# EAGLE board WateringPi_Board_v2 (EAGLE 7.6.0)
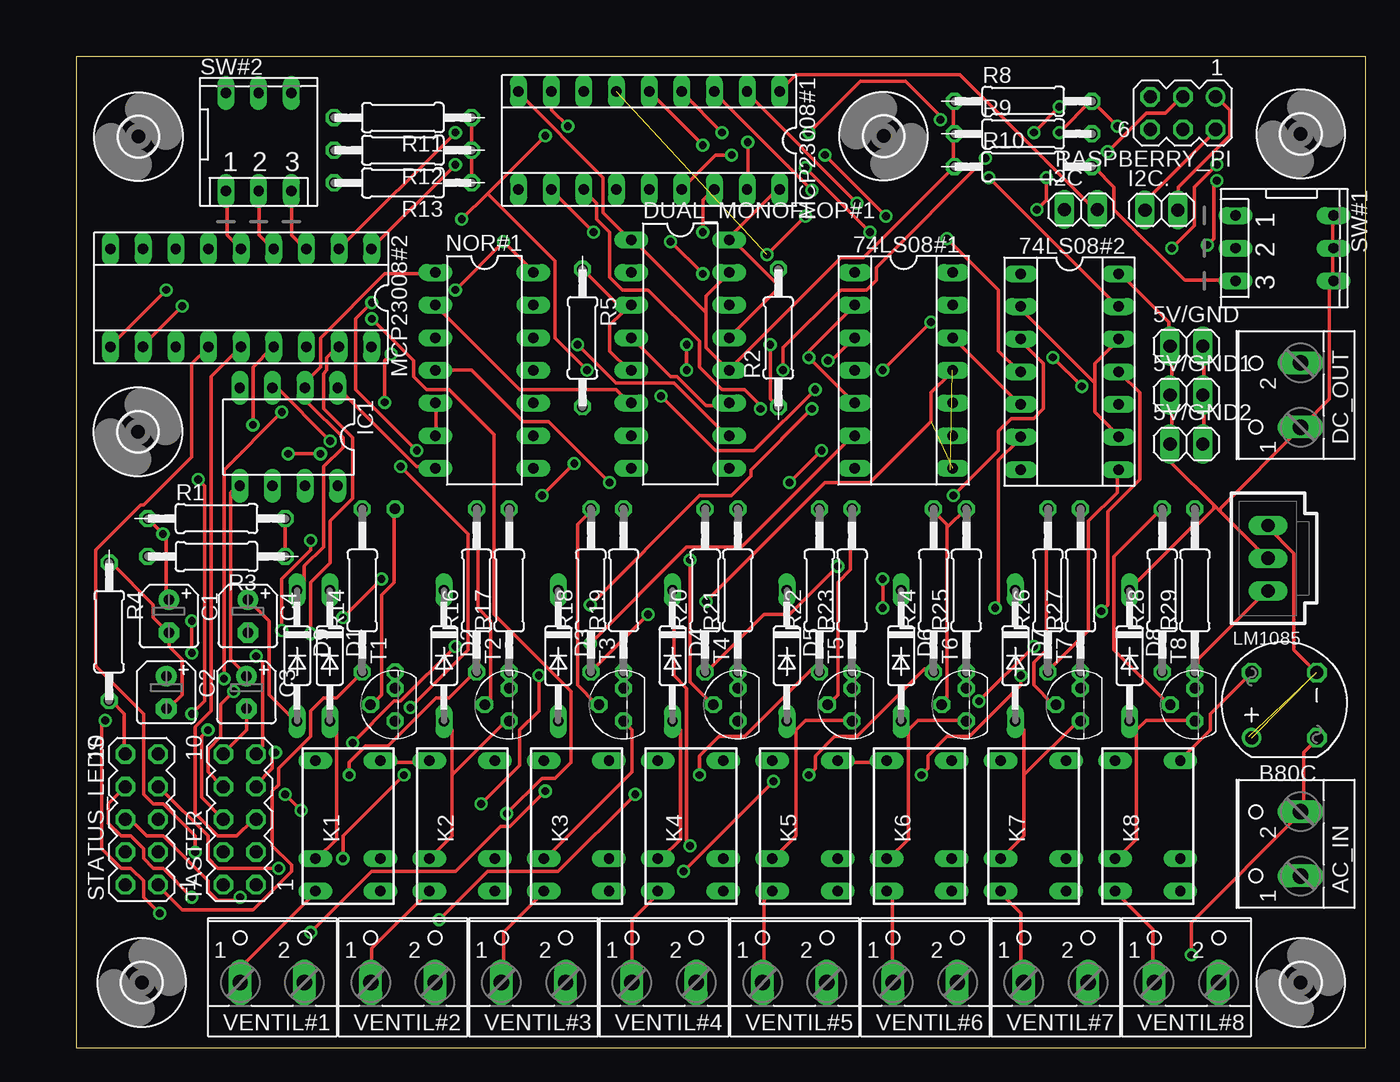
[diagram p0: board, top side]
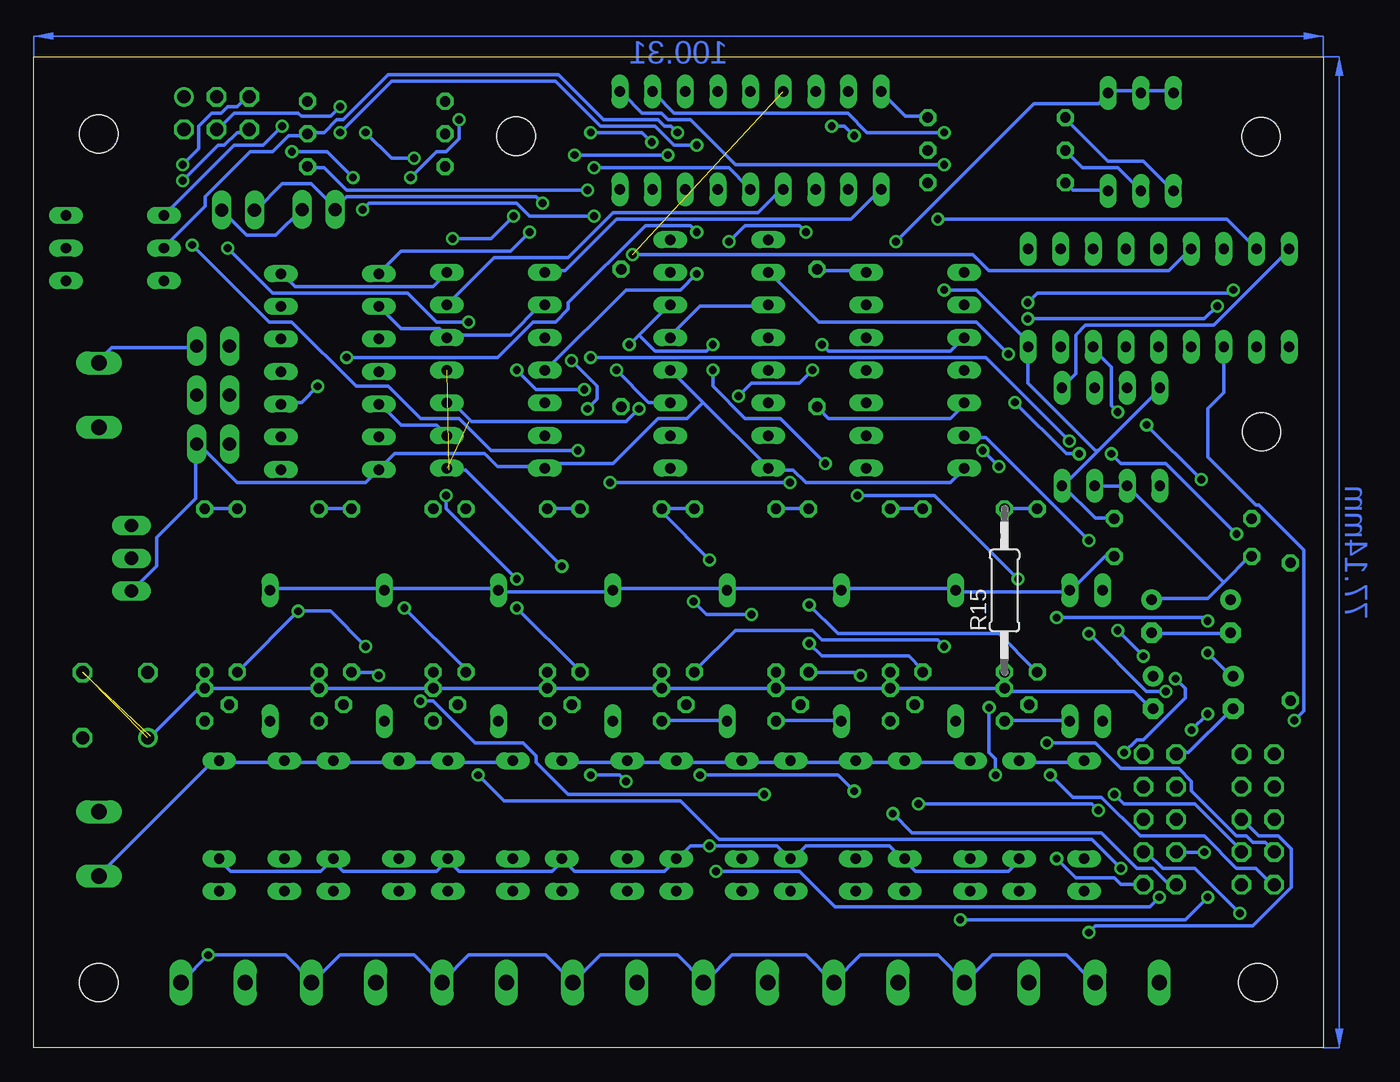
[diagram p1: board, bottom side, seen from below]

Size 100.31 x 77.14 mm. Coordinates in mm from the lower left corner, seen from the top.
Outline: 0,0 100.31,0 100.31,77.14 0,77.14 0,0
Copper layers (1*16): Top 0.035mm / dielectric 1.5mm / Bottom 0.035mm
Design rules "default": minimum track width 10mil, minimum drill 24mil, track to track 8mil, track to pad 8mil, pad to pad 8mil, via to via 8mil, smd to smd 8mil, copper to edge 40mil, drill to drill 8mil, minimum pad ring 10mil, minimum via ring 8mil, stop-mask expansion 4mil, vias tented up to drill 0mil, thermal gap 10mil

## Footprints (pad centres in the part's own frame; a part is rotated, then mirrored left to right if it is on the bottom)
1X02 = drill 1.016 long: 1 -1.27,0; 2 1.27,0
SOCKET-14 = drill 0.813 long: 1 -7.62,-3.81; 2 -5.08,-3.81; 3 -2.54,-3.81; 4 0,-3.81; 5 2.54,-3.81; 6 5.08,-3.81; 7 7.62,-3.81; 8 7.62,3.81; 9 5.08,3.81; 10 2.54,3.81; 11 0,3.81; 12 -2.54,3.81; 13 -5.08,3.81; 14 -7.62,3.81
W237-102 = drill 1.194 long: 1 -2.5,-1.27; 2 2.5,-1.27
RB1A = drill 1.016: + -2.54,2.54 | drill 1.016 octagon: - 2.54,-2.54; AC1 2.54,2.54; AC2 -2.54,-2.54
B45181A = drill 0.813 pad 1.6: + -1.27,0 | drill 0.813 pad 1.6 octagon: - 1.27,0
DO35-10 = drill 0.813 long: A 5.08,0; C -5.08,0
DIL16 = drill 0.813 long: 1 -8.89,-3.81; 2 -6.35,-3.81; 3 -3.81,-3.81; 4 -1.27,-3.81; 5 1.27,-3.81; 6 3.81,-3.81; 7 6.35,-3.81; 8 8.89,-3.81; 9 8.89,3.81; 10 6.35,3.81; 11 3.81,3.81; 12 1.27,3.81; 13 -1.27,3.81; 14 -3.81,3.81; 15 -6.35,3.81; 16 -8.89,3.81
3,0 = hole 3: 0,0
DIL-08 = drill 0.813 long: 1 -3.81,-3.81; 2 -1.27,-3.81; 3 1.27,-3.81; 4 3.81,-3.81; 5 3.81,3.81; 6 1.27,3.81; 7 -1.27,3.81; 8 -3.81,3.81
G5V1 = drill 0.813 long: 1 -5.08,-2.54; 2 -2.54,-2.54; 5 5.08,-2.54; 6 5.08,2.54; 9 -2.54,2.54; 10 -5.08,2.54
70543-03 = drill 1.016 long: 1 -2.54,0; 2 0,0; 3 2.54,0
SOCKET-18 = drill 0.813 long: 1 -10.16,-3.81; 2 -7.62,-3.81; 3 -5.08,-3.81; 4 -2.54,-3.81; 5 0,-3.81; 6 2.54,-3.81; 7 5.08,-3.81; 8 7.62,-3.81; 9 10.16,-3.81; 10 10.16,3.81; 11 7.62,3.81; 12 5.08,3.81; 13 2.54,3.81; 14 0,3.81; 15 -2.54,3.81; 16 -5.08,3.81; 17 -7.62,3.81; 18 -10.16,3.81
DIL14 = drill 0.813 long: 1 -7.62,-3.81; 2 -5.08,-3.81; 3 -2.54,-3.81; 4 0,-3.81; 5 2.54,-3.81; 6 5.08,-3.81; 7 7.62,-3.81; 8 7.62,3.81; 9 5.08,3.81; 10 2.54,3.81; 11 0,3.81; 12 -2.54,3.81; 13 -5.08,3.81; 14 -7.62,3.81
9/1 = drill 0.813 octagon: 1 -5.35,0; 2 5.35,0
0207/12 = drill 0.813 octagon: 1 -6.35,0; 2 6.35,0
MA03-2 = drill 1.016: 1 -2.54,-1.27 | drill 1.016 octagon: 2 -2.54,1.27; 3 0,-1.27; 4 0,1.27; 5 2.54,-1.27; 6 2.54,1.27
MA05-2 = drill 1.016 octagon: 1 -5.08,-1.27; 2 -5.08,1.27; 3 -2.54,-1.27; 4 -2.54,1.27; 5 0,-1.27; 6 0,1.27; 7 2.54,-1.27; 8 2.54,1.27; 9 5.08,-1.27; 10 5.08,1.27
DP-03 = drill 0.813 long: 1 -2.54,-3.81; 2 0,-3.81; 3 2.54,-3.81; 4 2.54,3.81; 5 0,3.81; 6 -2.54,3.81
TO92 = drill 0.813 octagon: 1 1.27,0; 2 0,1.905; 3 -1.27,0

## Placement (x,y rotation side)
5V/GND  [1X02]  86.36,54.61 0 top
5V/GND1  [1X02]  86.36,50.8 0 top
5V/GND2  [1X02]  86.36,46.99 0 top
74LS08#1  [SOCKET-14]  64.36,52.72 270 top
74LS08#2  [SOCKET-14]  77.26,52.62 270 top
AC_IN  [W237-102]  93.98,15.88 90 top
B80C  RECTIFIER-RB1A  [RB1A]  93.98,26.67 90 top
C1  10uF  [B45181A]  7.19,33.59 270 top
C2  10uF  [B45181A]  6.99,27.65 270 top
C3  10nF  [B45181A]  13.23,27.65 270 top
C4  10uF  [B45181A]  13.34,33.59 270 top
D1  1N4148DO35-10  [DO35-10]  19.7,30.52 270 top
D2  1N4148DO35-10  [DO35-10]  28.59,30.52 270 top
D3  1N4148DO35-10  [DO35-10]  37.48,30.52 270 top
D4  1N4148DO35-10  [DO35-10]  46.37,30.52 270 top
D5  1N4148DO35-10  [DO35-10]  55.26,30.52 270 top
D6  1N4148DO35-10  [DO35-10]  64.15,30.52 270 top
D7  1N4148DO35-10  [DO35-10]  73.04,30.52 270 top
D8  1N4148DO35-10  [DO35-10]  81.93,30.52 270 top
D9  1N4148DO35-10  [DO35-10]  17.16,30.52 270 top
DC_OUT  [W237-102]  93.98,50.8 90 top
DUAL_MONOFLOP#1  4538N  [DIL16]  46.99,53.99 270 top
H1  RPI-HOLE3.0  [3,0]  4.83,70.91 0 top
H2  RPI-HOLE3.0  [3,0]  62.8,70.94 270 top
H5  MOUNT-HOLE3.0  [3,0]  4.78,47.94 0 top
H6  MOUNT-HOLE3.0  [3,0]  5.08,5.08 0 top
H7  MOUNT-HOLE3.0  [3,0]  95.25,71.12 0 top
H8  MOUNT-HOLE3.0  [3,0]  95.25,5.08 0 top
I2C  [1X02]  78.15,65.24 0 top
I2C.  [1X02]  84.41,65.2 0 top
IC1  NE555  [DIL-08]  16.51,47.54 180 top
K1  G5V1  [G5V1]  21.12,17.27 90 top
K2  G5V1  [G5V1]  30.01,17.27 90 top
K3  G5V1  [G5V1]  38.9,17.27 90 top
K4  G5V1  [G5V1]  47.79,17.27 90 top
K5  G5V1  [G5V1]  56.68,17.27 90 top
K6  G5V1  [G5V1]  65.57,17.27 90 top
K7  G5V1  [G5V1]  74.46,17.27 90 top
K8  G5V1  [G5V1]  83.35,17.27 90 top
LM1085  C-GRID-03-70543  [70543-03]  92.71,38.1 90 top
MCP23008#1  [SOCKET-18]  44.55,70.61 180 top
MCP23008#2  [SOCKET-18]  12.8,58.35 180 top
NOR#1  7402N  [DIL14]  31.75,52.72 270 top
R1  1M  [9/1]  10.9,41.19 0 top
R2  1M  [9/1]  54.61,55.24 90 top
R3  1M  [9/1]  10.9,38.24 180 top
R4  Null Ohm  [9/1]  2.54,32.38 270 top
R5  1M  [9/1]  39.37,55.24 270 top
R8  1M  [9/1]  73.66,73.66 0 top
R9  1M  [9/1]  73.66,71.12 0 top
R10  1M  [9/1]  73.66,68.58 0 top
R11  1M  [9/1]  25.4,72.39 180 top
R12  1M  [9/1]  25.4,69.85 180 top
R13  1M  [9/1]  25.4,67.31 180 top
R14  2,2k  [0207/12]  22.24,35.6 90 top
R15  2,2k  [0207/12]  24.78,35.6 90 bottom
R16  2,2k  [0207/12]  31.13,35.6 90 top
R17  2,2k  [0207/12]  33.67,35.6 90 top
R18  2,2k  [0207/12]  40.02,35.6 90 top
R19  2,2k  [0207/12]  42.56,35.6 90 top
R20  2,2k  [0207/12]  48.91,35.6 90 top
R21  2,2k  [0207/12]  51.45,35.6 90 top
R22  2,2k  [0207/12]  57.8,35.6 90 top
R23  2,2k  [0207/12]  60.34,35.6 90 top
R24  2,2k  [0207/12]  66.69,35.6 90 top
R25  2,2k  [0207/12]  69.23,35.6 90 top
R26  2,2k  [0207/12]  75.58,35.6 90 top
R27  2,2k  [0207/12]  78.12,35.6 90 top
R28  2,2k  [0207/12]  84.47,35.6 90 top
R29  2,2k  [0207/12]  87.01,35.6 90 top
RASPBERRY_PI  [MA03-2]  86.09,72.74 180 top
STATUS_LEDS  [MA05-2]  5.08,17.78 90 top
SW#1  [DP-03]  93.98,62.23 270 top
SW#2  [DP-03]  14.18,70.5 0 top
T1  BC337  [TO92]  24.78,26.71 90 top
T2  BC337  [TO92]  33.67,26.71 90 top
T3  BC337  [TO92]  42.56,26.71 90 top
T4  BC337  [TO92]  51.45,26.71 90 top
T5  BC337  [TO92]  60.34,26.71 90 top
T6  BC337  [TO92]  69.23,26.71 90 top
T7  BC337  [TO92]  78.12,26.71 90 top
T8  BC337  [TO92]  87.01,26.71 90 top
TASTER  [MA05-2]  12.7,17.78 90 top
VENTIL#1  [W237-102]  15.24,6.35 0 top
VENTIL#2  [W237-102]  25.4,6.35 0 top
VENTIL#3  [W237-102]  35.56,6.35 0 top
VENTIL#4  [W237-102]  45.72,6.35 0 top
VENTIL#5  [W237-102]  55.88,6.35 0 top
VENTIL#6  [W237-102]  66.04,6.35 0 top
VENTIL#7  [W237-102]  76.2,6.35 0 top
VENTIL#8  [W237-102]  86.36,6.35 0 top

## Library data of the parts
5V/GND 5V/GND1 5V/GND2 I2C I2C. = pinhead
74LS08#1 74LS08#2 MCP23008#1 MCP23008#2 = ic-package
AC_IN DC_OUT VENTIL#1-VENTIL#8 = con-wago-500; MPN: 237-102; OC_FARNELL: unknown; OC_NEWARK: 70K9898
B80C = rectifier
C1-C4 R14-R29 = resistor
D1-D9 = diode
DUAL_MONOFLOP#1 = 45xx
H1 H2 H5-H8 = holes
IC1 = st-microelectronics; MF: Arrow Electronics; MPN: NE555N; OC_FARNELL: 1467742; OC_NEWARK: 89K1486
K1-K8 = relay
LM1085 = con-molex; OC_FARNELL: unknown; OC_NEWARK: unknown
NOR#1 = 74ttl-din
R1-R5 R8-R13 = customize
RASPBERRY_PI STATUS_LEDS TASTER = con-lstb; OC_FARNELL: unknown; OC_NEWARK: unknown
SW#1 SW#2 = switch-dil; MPN: MCDP03; OC_FARNELL: 1522004; OC_NEWARK: 74M2976
T1-T8 = transistor

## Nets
+5V: 5V/GND1.1 5V/GND2.1 5V/GND.1 74LS08#1.14 74LS08#2.14 D1.C D2.C D3.C D4.C D5.C D6.C D7.C D8.C DC_OUT.1 DUAL_MONOFLOP#1.3 DUAL_MONOFLOP#1.5 DUAL_MONOFLOP#1.13 DUAL_MONOFLOP#1.16 IC1.4 IC1.8 K1.2 K2.2 K3.2 K4.2 K5.2 K6.2 K7.2 K8.2 LM1085.2 MCP23008#1.18 MCP23008#2.18 NOR#1.14 R1.2 R2.2 R3.1 R5.1 SW#1.4 SW#1.5 SW#1.6 SW#2.4 SW#2.5 SW#2.6
AC_1/2: AC_IN.1 B80C.AC1 K1.5 K1.6 K2.5 K2.6 K3.5 K3.6 K4.5 K4.6 K5.5 K5.6 K6.5 K6.6 K7.5 K7.6 K8.5 K8.6
AC_2/2: AC_IN.2 B80C.AC2 VENTIL#1.2 VENTIL#2.2 VENTIL#3.2 VENTIL#4.2 VENTIL#5.2 VENTIL#6.2 VENTIL#7.2 VENTIL#8.2
GND: 5V/GND1.2 5V/GND2.2 5V/GND.2 74LS08#1.7 74LS08#2.7 B80C.- C1.- C2.- C3.- C4.- DC_OUT.2 DUAL_MONOFLOP#1.1 DUAL_MONOFLOP#1.8 DUAL_MONOFLOP#1.12 DUAL_MONOFLOP#1.15 IC1.1 LM1085.1 MCP23008#1.9 MCP23008#2.9 NOR#1.7 R4.1 R8.1 R9.1 R10.1 R11.1 R12.1 R13.1 R15.1 R17.1 R19.1 R21.1 R23.1 R25.1 R27.1 R29.1 T1.1 T2.1 T3.1 T4.1 T5.1 T6.1 T7.1 T8.1 TASTER.10
I2C_SCL: I2C.2 I2C..2 MCP23008#1.1 MCP23008#2.1 RASPBERRY_PI.1
I2C_SDA: I2C.1 I2C..1 MCP23008#1.2 MCP23008#2.2 RASPBERRY_PI.2
INTERRUPT: MCP23008#2.8 RASPBERRY_PI.5
IS_ALIVE: D9.C IC1.2 NOR#1.1
KEEP_ALIVE: DUAL_MONOFLOP#1.4 DUAL_MONOFLOP#1.11 RASPBERRY_PI.4
MCP23008#1_A0: MCP23008#1.5 R8.2 SW#1.1
MCP23008#1_A1: MCP23008#1.4 R9.2 SW#1.2
MCP23008#1_A2: MCP23008#1.3 R10.2 SW#1.3
MCP23008#1_OUT0: 74LS08#1.1 MCP23008#1.10
MCP23008#1_OUT1: 74LS08#1.4 MCP23008#1.11
MCP23008#1_OUT2: 74LS08#1.10 MCP23008#1.12
MCP23008#1_OUT3: 74LS08#1.13 MCP23008#1.13
MCP23008#1_OUT4: 74LS08#2.1 MCP23008#1.14
MCP23008#1_OUT5: 74LS08#2.4 MCP23008#1.15
MCP23008#1_OUT6: 74LS08#2.10 MCP23008#1.16
MCP23008#1_OUT7: 74LS08#2.13 MCP23008#1.17
MCP23008#2_A0: MCP23008#2.5 R11.2 SW#2.1
MCP23008#2_A1: MCP23008#2.4 R12.2 SW#2.2
MCP23008#2_A2: MCP23008#2.3 R13.2 SW#2.3
MCP_RESET: MCP23008#1.6 MCP23008#2.6 RASPBERRY_PI.3
N$1: R14.2 R15.2 T1.2
N$2: C2.+ DUAL_MONOFLOP#1.14 R2.1
N$3: C1.+ DUAL_MONOFLOP#1.2 R1.1
N$4: DUAL_MONOFLOP#1.10 NOR#1.3
N$5: DUAL_MONOFLOP#1.6 NOR#1.2
N$6: R16.2 R17.2 T2.2
N$7: C3.+ IC1.5
N$8: D1.A K1.9 T1.3
N$9: D2.A K2.9 T2.3
N$10: R18.2 R19.2 T3.2
N$11: D3.A K3.9 T3.3
N$12: B80C.+ LM1085.3
N$13: R20.2 R21.2 T4.2
N$14: R4.2 STATUS_LEDS.10
N$15: C4.+ D9.A IC1.6 IC1.7 R3.2
N$22: D4.A K4.9 T4.3
N$23: R22.2 R23.2 T5.2
N$24: D5.A K5.9 T5.3
N$25: R24.2 R25.2 T6.2
N$26: D6.A K6.9 T6.3
N$27: R26.2 R27.2 T7.2
N$28: D7.A K7.9 T7.3
N$29: R28.2 R29.2 T8.2
N$30: D8.A K8.9 T8.3
NOTAUS: NOR#1.4 RASPBERRY_PI.6
NOTAUS_RAW: NOR#1.5 NOR#1.6 R5.2 TASTER.9
RELAIS#1_ENABLE: 74LS08#1.3 R14.1 STATUS_LEDS.1
RELAIS#1_OUT: K1.10 VENTIL#1.1
RELAIS#2_ENABLE: 74LS08#1.6 R16.1 STATUS_LEDS.2
RELAIS#2_OUT: K2.10 VENTIL#2.1
RELAIS#3_ENABLE: 74LS08#1.8 R18.1 STATUS_LEDS.3
RELAIS#3_OUT: K3.10 VENTIL#3.1
RELAIS#4_ENABLE: 74LS08#1.11 R20.1 STATUS_LEDS.4
RELAIS#4_OUT: K4.10 VENTIL#4.1
RELAIS#5_ENABLE: 74LS08#2.3 R22.1 STATUS_LEDS.5
RELAIS#5_OUT: K5.10 VENTIL#5.1
RELAIS#6_ENABLE: 74LS08#2.6 R24.1 STATUS_LEDS.6
RELAIS#6_OUT: K6.10 VENTIL#6.1
RELAIS#7_ENABLE: 74LS08#2.8 R26.1 STATUS_LEDS.7
RELAIS#7_OUT: K7.10 VENTIL#7.1
RELAIS#8_ENABLE: 74LS08#2.11 R28.1 STATUS_LEDS.8
RELAIS#8_OUT: K8.10 VENTIL#8.1
RPI_STILL_ALIVE: 74LS08#1.2 74LS08#1.5 74LS08#1.9 74LS08#1.12 74LS08#2.2 74LS08#2.5 74LS08#2.9 74LS08#2.12 IC1.3
TASTE#1: MCP23008#2.10 TASTER.1
TASTE#2: MCP23008#2.11 TASTER.2
TASTE#3: MCP23008#2.12 TASTER.3
TASTE#4: MCP23008#2.13 TASTER.4
TASTE#5: MCP23008#2.14 TASTER.5
TASTE#6: MCP23008#2.15 TASTER.6
TASTE#7: MCP23008#2.16 TASTER.7
TASTE#8: MCP23008#2.17 TASTER.8

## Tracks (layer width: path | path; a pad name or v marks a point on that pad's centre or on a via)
+5V  (via drill 0.61)
  Top 0.254: 54.48,59.48 54.48,60.48 R2.2 | 54.48,59.48 54.48,58.98 50.98,55.48 DUAL_MONOFLOP#1.13 | 54.48,59.48 50.98,62.98 | 50.98,62.98 50.98,63.23 54.48,66.73 MCP23008#1.18 | 50.98,62.98 DUAL_MONOFLOP#1.16 | 42.48,57.23 42.98,57.73 DUAL_MONOFLOP#1.3 42.48,57.23 | 42.48,57.23 41.48,56.23 41.48,54.23 42.98,52.73 DUAL_MONOFLOP#1.5 | 42.48,57.23 42.48,57.48 39.48,60.48 R5.1 | NOR#1.14 35.48,60.48 v33.23,62.73 v29.48,58.98 | 74LS08#2.14 81.23,60.23 84.98,56.48 84.98,54.73 5V/GND.1 85.23,54.48 85.23,50.98 5V/GND1.1 85.23,50.73 85.23,47.23 5V/GND2.1 85.23,46.98 85.23,45.48 88.48,42.23 | 97.73,62.23 97.73,59.73 SW#1.4 97.73,59.48 97.48,59.23 97.48,50.48 95.48,48.48 DC_OUT.1 95.23,48.23 88.98,41.98 88.98,41.73 | 97.73,62.23 97.73,64.73 SW#1.6 | 97.73,62.23 SW#1.5 | 88.48,42.23 88.98,41.73 | 88.98,41.73 92.48,38.23 LM1085.2 | 88.48,42.23 88.48,41.98 87.23,40.73 86.98,40.73 81.98,35.73 D8.C | R1.2 16.23,40.98 16.23,38.48 R3.1 | v47.73,15.73 47.48,15.98 47.48,27.98 46.48,28.98 46.48,35.48 D4.C
  Bottom 0.254: SW#2.6 11.73,74.48 13.98,74.48 SW#2.5 14.23,74.48 16.48,74.48 SW#2.4 16.73,74.23 17.48,73.48 22.48,73.48 v33.23,62.73 | NOR#1.14 35.73,60.48 39.23,60.48 R5.1 | DUAL_MONOFLOP#1.13 50.73,55.48 48.48,57.73 43.23,57.73 DUAL_MONOFLOP#1.3 | K1.2 23.73,14.48 24.48,13.73 31.73,13.73 32.48,14.48 K2.2 32.73,14.73 33.73,15.73 40.23,15.73 41.23,14.73 K3.2 41.48,14.73 42.48,15.73 v47.73,15.73 49.23,15.73 50.23,14.73 K4.2 50.48,14.48 51.23,13.73 58.23,13.73 58.98,14.48 K5.2 59.23,14.48 59.98,13.73 67.23,13.73 67.98,14.48 K6.2 68.23,14.48 68.98,13.73 76.23,13.73 76.98,14.48 K7.2 77.23,14.48 77.98,13.73 84.98,13.73 85.73,14.48 K8.2 | 74LS08#1.14 68.23,60.23 69.23,59.23 79.98,59.23 80.98,60.23 74LS08#2.14 | D8.C 81.73,35.73 73.23,35.73 D7.C 72.98,35.73 64.23,35.73 D6.C 63.98,35.48 55.48,35.48 D5.C 55.23,35.73 46.48,35.73 D4.C 46.23,35.73 37.73,35.73 D3.C 37.48,35.73 28.73,35.73 D2.C 28.48,35.48 19.73,35.48 D1.C 19.48,35.73 16.98,38.23 16.48,38.23 R3.1 | R1.2 16.48,41.23 17.73,41.23 20.23,43.73 IC1.8 20.23,43.98 19.98,43.98 17.48,46.48 | 17.48,46.48 12.73,51.23 IC1.4 | 17.48,46.48 17.73,46.48 22.98,51.73 22.98,54.48 MCP23008#2.18 22.73,54.73 26.98,58.98 v29.48,58.98
AC_1/2
  Top 0.254: B80C.AC1 91.23,28.98 88.23,25.98 88.23,24.73 85.98,22.48 K8.5 | K2.6 27.23,22.23 23.73,22.23 K1.5 | K5.5 59.23,22.23 62.98,22.23 K6.6
  Bottom 0.254: AC_IN.1 95.23,13.48 86.48,22.23 85.98,22.23 K8.5 85.73,22.23 80.98,22.23 K8.6 80.73,22.23 77.23,22.23 K7.5 76.98,22.23 71.98,22.23 K7.6 71.73,22.23 68.23,22.23 K6.5 67.98,22.23 63.23,22.23 K6.6 | K1.6 18.73,22.23 23.48,22.23 K1.5 | K5.5 58.98,22.23 54.23,22.23 K5.6 53.98,22.23 50.48,22.23 K4.5 50.23,22.23 45.48,22.23 K4.6 45.23,22.23 41.48,22.23 K3.5 41.23,22.23 36.48,22.23 K3.6 36.23,22.23 32.73,22.23 K2.5 32.48,22.23 27.48,22.23 K2.6
AC_2/2  (via drill 0.61)
  Top 0.254: B80C.AC2 96.48,23.98 95.48,22.98 95.48,18.48 AC_IN.2 95.23,18.23 86.73,9.73 v86.73,7.23
  Bottom 0.254: VENTIL#1.2 17.98,5.23 19.98,7.23 25.73,7.23 27.73,5.23 VENTIL#2.2 27.98,5.23 29.98,7.23 35.98,7.23 37.98,5.23 VENTIL#3.2 38.23,5.23 40.23,7.23 45.98,7.23 47.98,5.23 VENTIL#4.2 48.23,5.23 50.23,7.23 56.23,7.23 VENTIL#5.2 58.48,5.23 60.48,7.23 66.48,7.23 68.48,5.23 VENTIL#6.2 68.73,5.23 70.73,7.23 76.48,7.23 78.48,5.23 VENTIL#7.2 78.73,5.23 80.73,7.23 v86.73,7.23 88.73,5.23 VENTIL#8.2
GND  (1 unrouted)
  Top 0.254: NOR#1.7 27.73,45.23 26.48,45.23 20.48,51.23 IC1.1 | R13.1 30.73,67.48 30.73,69.73 R12.1 30.73,69.98 30.73,72.23 R11.1 | R8.1 68.23,73.48 68.23,71.23 R9.1 68.23,70.98 68.23,68.73 R10.1 68.23,68.48 61.23,61.48 59.48,61.48 50.98,52.98 50.98,52.73 DUAL_MONOFLOP#1.12 50.73,52.73 48.98,54.48 48.98,57.23 | 48.98,57.23 48.98,58.48 50.73,60.23 DUAL_MONOFLOP#1.15 | 48.98,57.23 43.23,62.98 DUAL_MONOFLOP#1.1 42.98,62.98 40.98,64.98 40.98,67.73 34.48,74.23 MCP23008#1.9 | TASTER.10 11.48,22.98 13.23,24.73 13.23,26.23 C3.- | R4.1 2.73,37.73 5.98,34.48 5.98,33.48 6.98,32.48 C1.- 7.23,32.23 7.23,31.23 8.23,30.23 8.23,27.48 7.23,26.48 C2.- | T1.1 24.73,27.98 24.73,29.23 R15.1 | T2.1 33.73,27.98 33.73,29.23 R17.1 | T3.1 42.48,27.98 42.48,29.23 R19.1 | T4.1 51.48,27.98 51.48,29.23 R21.1 | T7.1 78.23,27.98 78.23,29.23 R27.1 | T5.1 60.48,27.98 60.48,29.23 R23.1 | T6.1 69.23,29.23 R25.1 | 5V/GND2.2 87.73,47.23 87.73,50.73 5V/GND1.2 87.73,50.98 87.73,54.48 5V/GND.2 | T8.1 86.98,27.98 86.98,29.23 R29.1 87.23,29.48 87.23,30.23 92.48,35.48 LM1085.1
  Bottom 0.254: MCP23008#2.9 2.73,61.98 8.48,56.23 18.48,56.23 19.23,55.48 19.23,52.48 20.23,51.48 IC1.1 | MCP23008#1.9 34.23,74.23 32.48,72.48 30.98,72.48 R11.1 | 48.23,50.23 50.48,52.48 50.73,52.48 DUAL_MONOFLOP#1.12 | 48.23,50.23 43.23,45.23 DUAL_MONOFLOP#1.8 42.98,44.98 41.23,44.98 40.23,43.98 28.98,43.98 27.98,44.98 NOR#1.7 | 48.23,50.23 49.48,48.98 51.73,48.98 55.23,45.48 60.23,45.48 60.48,45.23 74LS08#1.7 60.73,45.23 64.23,45.23 65.23,46.23 72.23,46.23 73.23,45.23 74LS08#2.7 73.48,44.98 74.48,43.98 84.48,43.98 87.48,46.98 5V/GND2.2 87.73,46.98 87.73,42.73 90.73,39.73 90.73,37.48 92.48,35.73 LM1085.1 | C2.- 7.23,26.23 10.48,22.98 11.23,22.98 TASTER.10 | C4.- 13.23,32.23 7.23,32.23 C1.- | C3.- 13.48,26.48 14.73,27.73 24.73,27.73 T1.1 24.98,27.98 33.48,27.98 T2.1 33.73,27.98 42.48,27.98 T3.1 42.73,27.98 51.23,27.98 T4.1 51.48,27.98 60.23,27.98 T5.1 60.48,27.98 T6.1 69.48,27.98 77.98,27.98 T7.1 78.23,27.98 86.98,27.98 T8.1 87.23,27.73 87.73,27.73 91.23,24.23 | DC_OUT.2 95.23,53.48 94.23,54.48 87.73,54.48 5V/GND.2
I2C_SCL  (via drill 0.61)
  Top 0.254: RASPBERRY_PI.1 88.73,73.98 89.73,72.98 89.73,70.98 85.73,66.98 85.73,65.23 I2C..2 | v29.48,68.73 22.98,62.23 MCP23008#2.1 | I2C.2 79.23,65.23 68.73,75.73 55.98,75.73 54.73,74.48 MCP23008#1.1
  Bottom 0.254: I2C..2 85.48,64.98 83.73,63.23 81.48,63.23 79.48,65.23 I2C.2 | v29.48,68.73 45.73,68.73 49.23,72.23 50.98,72.23 51.48,72.73 52.98,72.73 54.48,74.23 MCP23008#1.1
I2C_SDA  (via drill 0.61)
  Top 0.254: RASPBERRY_PI.2 88.48,71.23 83.23,65.98 83.23,65.23 I2C..1 | v29.48,71.23 20.48,62.23 MCP23008#2.2 | v60.73,65.73 52.23,74.23 MCP23008#1.2
  Bottom 0.254: I2C..1 82.98,65.23 80.98,67.23 78.73,67.23 76.98,65.48 I2C.1 76.73,65.48 75.98,66.23 61.23,66.23 v60.73,65.73 | v29.48,71.23 35.48,71.23 36.98,72.73 50.48,72.73 51.98,74.23 MCP23008#1.2
INTERRUPT  (via drill 0.61)
  Top 0.254: v36.48,70.98 31.98,66.48 | 31.98,66.48 v29.98,64.48 | v38.23,71.73 36.98,72.98 36.98,74.23 | v88.73,68.73 86.98,66.98 86.98,63.98 v85.23,62.23 | v62.73,52.73 v66.48,56.48 | v57.48,51.23 52.73,46.48 49.73,46.48 v45.48,50.73 | v39.73,52.73 37.23,55.23 37.23,61.23 31.98,66.48
  Bottom 0.254: v29.98,64.48 7.48,64.48 5.23,62.23 MCP23008#2.8 | v36.48,70.98 37.23,71.73 v38.23,71.73 | v88.73,68.73 87.48,69.98 87.48,71.73 86.48,72.73 85.73,72.73 85.23,73.23 84.48,73.23 83.73,73.98 RASPBERRY_PI.5 | v85.23,62.23 81.73,58.73 71.23,58.73 68.98,56.48 v66.48,56.48 | v62.73,52.73 61.23,51.23 v57.48,51.23 | v45.48,50.73 44.48,51.73 40.73,51.73 v39.73,52.73
IS_ALIVE
  Top 0.254: D9.C 17.23,35.73 17.73,36.23 17.73,37.48 19.23,38.98 19.23,45.23 20.73,46.73 20.73,47.48 17.98,50.23 17.98,51.23 IC1.2 17.98,51.48 17.98,51.98 18.98,52.98 18.98,55.23 23.98,60.23 27.73,60.23 NOR#1.1
KEEP_ALIVE  (via drill 0.61)
  Top 0.254: DUAL_MONOFLOP#1.4 43.23,55.23 46.23,52.23 46.73,52.23 48.98,49.98 50.73,49.98 DUAL_MONOFLOP#1.11 | v74.48,71.23 v76.48,73.23 | v70.73,69.23 62.23,60.73 62.23,59.73 61.48,58.98 59.48,58.98 54.98,54.48 v54.98,52.73
  Bottom 0.254: v76.48,73.23 77.23,72.48 79.48,72.48 79.73,72.73 84.73,72.73 85.98,71.48 RASPBERRY_PI.4 | v74.48,71.23 72.48,69.23 v70.73,69.23 | v54.98,52.73 52.48,50.23 50.98,50.23 DUAL_MONOFLOP#1.11
MCP23008#1_A0  (via drill 0.61)
  Top 0.254: v48.73,70.23 44.73,74.23 MCP23008#1.5 | v76.48,71.23 78.98,73.73 R8.2 79.23,73.48 v80.98,71.73
  Bottom 0.254: v48.73,70.23 50.48,70.23 51.98,71.73 56.23,71.73 59.73,75.23 72.48,75.23 v76.48,71.23 | v80.98,71.73 82.48,70.23 84.73,70.23 89.98,64.98 SW#1.1
MCP23008#1_A1  (via drill 0.61)
  Top 0.254: v50.23,71.23 47.23,74.23 MCP23008#1.4
  Bottom 0.254: v50.23,71.23 50.73,71.73 51.23,71.73 51.73,72.23 55.98,72.23 59.48,75.73 72.73,75.73 76.23,72.23 76.73,72.23 77.73,71.23 78.98,71.23 R9.2 79.23,70.98 80.48,70.98 81.73,69.73 83.48,69.73 86.98,66.23 86.98,65.48 90.23,62.23 SW#1.2
MCP23008#1_A2  (via drill 0.61)
  Top 0.254: v57.23,66.73 49.73,74.23 MCP23008#1.3 | SW#1.3 89.98,59.73 86.23,59.73 80.73,65.23 80.73,66.98 79.23,68.48 R10.2
  Bottom 0.254: v57.23,66.73 75.98,66.73 77.73,68.48 78.98,68.48 R10.2
MCP23008#1_OUT0
  Bottom 0.254: MCP23008#1.10 34.48,66.73 36.73,64.48 54.98,64.48 58.98,60.48 60.48,60.48 74LS08#1.1
MCP23008#1_OUT1  (via drill 0.61)
  Top 0.254: v40.23,63.48 36.98,66.73 MCP23008#1.11 | v48.73,60.23 v46.23,62.73
  Bottom 0.254: v40.23,63.48 40.73,63.98 44.98,63.98 v46.23,62.73 | v48.73,60.23 49.98,58.98 54.23,58.98 60.48,52.73 74LS08#1.4
MCP23008#1_OUT2  (via drill 0.61)
  Top 0.254: v53.23,49.73 53.23,49.98 51.98,51.23 50.23,51.23 48.48,52.98 48.48,54.98 44.48,58.98 42.48,58.98 41.48,59.98 41.48,63.48 40.48,64.48 40.48,65.73 39.48,66.73 MCP23008#1.12
  Bottom 0.254: v53.23,49.73 54.23,48.73 66.23,48.73 67.48,49.98 67.98,49.98 74LS08#1.10
MCP23008#1_OUT3
  Bottom 0.254: MCP23008#1.13 42.23,66.73 43.98,64.98 55.23,64.98 58.73,61.48 64.48,61.48 67.98,57.98 74LS08#1.13
MCP23008#1_OUT4  (via drill 0.61)
  Top 0.254: v61.73,63.48 v56.73,68.48
  Bottom 0.254: v56.73,68.48 46.23,68.48 44.73,66.98 MCP23008#1.14 | v61.73,63.48 63.23,61.98 71.73,61.98 73.23,60.48 74LS08#2.1
MCP23008#1_OUT5  (via drill 0.61)
  Top 0.254: v50.98,69.48 49.73,69.48 47.23,66.98 MCP23008#1.15 | v62.98,64.73 v58.23,69.48 | v67.73,62.98 71.73,58.98 71.73,54.23 73.23,52.73 74LS08#2.4
  Bottom 0.254: v58.23,69.48 v50.98,69.48 | v62.98,64.73 64.73,62.98 v67.73,62.98
MCP23008#1_OUT6  (via drill 0.61)
  Top 0.254: v48.73,63.48 48.73,65.98 49.48,66.73 MCP23008#1.16 | v78.23,51.48 v75.98,53.73
  Bottom 0.254: v48.73,63.48 49.23,63.98 52.73,63.98 58.73,57.98 58.73,57.48 59.73,56.48 61.48,56.48 64.23,53.73 v75.98,53.73 | v78.23,51.48 79.48,50.23 80.98,50.23 74LS08#2.10
MCP23008#1_OUT7  (via drill 0.61)
  Top 0.254: v52.23,70.48 52.23,66.98 MCP23008#1.17 | v56.98,71.23 60.98,75.23 64.48,75.23 67.23,72.48 v67.23,72.23 | v70.98,67.73 80.98,57.73 74LS08#2.13
  Bottom 0.254: v52.23,70.48 52.98,71.23 v56.98,71.23 | v67.23,72.23 67.23,70.73 68.23,69.73 68.98,69.73 v70.98,67.73
MCP23008#2_A0
  Top 0.254: MCP23008#2.5 12.73,62.23 11.73,63.23 11.73,66.48 SW#2.1
  Bottom 0.254: R11.2 19.98,72.23 16.73,68.98 13.98,68.98 11.73,66.73 SW#2.1
MCP23008#2_A1
  Top 0.254: MCP23008#2.4 15.23,62.23 14.23,63.23 14.23,66.48 SW#2.2
  Bottom 0.254: R12.2 19.98,69.73 18.73,68.48 15.98,68.48 14.23,66.73 SW#2.2
MCP23008#2_A2
  Top 0.254: MCP23008#2.3 17.73,62.23 16.73,63.23 16.73,66.48 SW#2.3
  Bottom 0.254: R13.2 19.98,67.23 19.48,66.73 16.73,66.73 SW#2.3
MCP_RESET  (via drill 0.61)  (1 unrouted)
  Top 0.254: v56.73,64.73 v53.73,61.73 | v74.73,65.23 75.48,65.98 v75.48,67.73 | v80.23,69.73 83.23,72.73 84.73,72.73 85.98,73.98 RASPBERRY_PI.3
  Bottom 0.254: v53.73,61.73 27.23,61.73 25.98,60.48 11.98,60.48 10.48,61.98 MCP23008#2.6 | v56.73,64.73 61.73,64.73 62.73,65.73 74.23,65.73 v74.73,65.23 | v75.48,67.73 77.48,69.73 v80.23,69.73
N$1
  Top 0.254: T1.2 22.98,26.73 23.73,27.48 23.73,35.23 24.73,36.23 24.73,41.73 R15.2
  Bottom 0.254: R14.2 22.48,41.98 24.73,41.98 R15.2
N$2  (via drill 0.61)
  Top 0.254: v53.98,54.73 53.98,50.48 54.48,49.98 R2.1 | v8.98,33.23 v8.98,30.73 | v23.73,36.48 v20.73,33.48 | v38.73,45.48 v36.23,42.98 | v47.48,54.73 v47.48,52.73
  Bottom 0.254: v53.98,54.73 53.23,55.48 | 53.23,55.48 50.98,57.73 DUAL_MONOFLOP#1.14 | v8.98,30.73 7.23,28.98 C2.+ | v8.98,33.23 9.23,33.48 v20.73,33.48 | v23.73,36.48 30.23,42.98 v36.23,42.98 | v38.73,45.48 42.23,48.98 44.98,48.98 47.48,51.48 v47.48,52.73 | v47.48,54.73 47.98,54.23 51.98,54.23 53.23,55.48
N$3  (via drill 0.61)
  Top 0.254: R1.1 5.73,40.98 v6.73,39.98 6.98,39.73 6.98,34.98 C1.+ | v24.48,53.98 23.98,53.48 v23.98,50.23 | v16.48,46.23 v18.98,46.23
  Bottom 0.254: v24.48,53.98 26.98,56.48 39.23,56.48 42.98,60.23 DUAL_MONOFLOP#1.2 | v23.98,50.23 19.98,46.23 v18.98,46.23 | v16.48,46.23 15.73,45.48 12.23,45.48 v6.73,39.98
N$4  (via drill 0.61)
  Top 0.254: v38.98,54.73 41.98,51.73 46.48,51.73 50.73,47.48 DUAL_MONOFLOP#1.10
  Bottom 0.254: v38.98,54.73 38.48,54.23 28.98,54.23 27.98,55.23 NOR#1.3
N$5
  Top 0.254: NOR#1.2 27.98,57.73 34.48,51.23 41.98,51.23 42.98,50.23 DUAL_MONOFLOP#1.6
N$6
  Top 0.254: T2.2 31.98,26.73 32.23,26.98 32.23,33.23 31.23,34.23 31.23,41.73 R16.2
  Bottom 0.254: R17.2 33.48,41.98 31.23,41.98 R16.2
N$7
  Top 0.254: IC1.5 12.48,43.73 11.98,43.23 11.98,30.23 13.23,28.98 C3.+
N$8
  Top 0.254: K1.9 18.73,14.73 20.23,16.23 20.23,24.73 19.73,25.23 D1.A
  Bottom 0.254: T1.3 24.73,25.48 19.73,25.48 D1.A
N$9
  Top 0.254: 29.23,21.23 29.23,24.73 28.73,25.23 D2.A | 29.23,21.23 29.23,16.48 K2.9 | 29.23,21.23 33.48,25.48 T2.3
N$10
  Top 0.254: T3.2 40.48,26.73 38.98,28.23 38.98,40.73 39.98,41.73 R18.2
  Bottom 0.254: R18.2 40.23,41.98 42.48,41.98 R19.2
N$11
  Top 0.254: K3.9 36.48,14.73 43.23,21.48 43.23,24.73 42.73,25.23 T3.3
  Bottom 0.254: D3.A 37.73,25.48 42.48,25.48 T3.3
N$12  (1 unrouted)
  Top 0.254: 96.48,29.23 94.73,30.98 94.73,38.48 92.73,40.48 LM1085.3
N$13  (via drill 0.61)
  Top 0.254: v47.73,37.98 47.73,28.48 49.48,26.73 T4.2
  Bottom 0.254: R20.2 48.98,41.98 51.23,41.98 R21.2 51.48,41.73 v47.73,37.98
N$14
  Top 0.254: R4.2 2.73,26.98 3.73,25.98 3.73,22.98 STATUS_LEDS.10
N$15
  Top 0.254: D9.A 16.98,25.48 14.98,27.48 14.98,33.23 13.48,34.73 C4.+
  Bottom 0.254: IC1.7 17.73,43.73 15.48,43.73 IC1.6 7.73,36.23 | 7.73,36.23 8.98,34.98 13.23,34.98 C4.+ | 7.73,36.23 5.73,38.23 R3.2
N$22
  Top 0.254: K4.9 45.48,14.73 46.98,16.23 46.98,24.73 46.48,25.23 D4.A
  Bottom 0.254: T4.3 51.23,25.48 46.48,25.48 D4.A
N$23
  Top 0.254: T5.2 58.48,26.73 59.23,27.48 59.23,36.23 60.23,37.23 60.23,41.73 R23.2
  Bottom 0.254: R22.2 57.98,41.98 60.23,41.98 R23.2
N$24
  Top 0.254: 55.98,24.73 55.98,16.48 54.23,14.73 K5.9 | 55.98,24.73 55.48,25.23 D5.A | 55.98,24.73 56.73,25.48 60.23,25.48 T5.3
N$25
  Top 0.254: 67.73,40.48 67.73,40.73 66.73,41.73 R24.2 | 67.73,40.48 67.73,26.98 67.48,26.73 T6.2 | 67.73,40.48 69.23,41.98 R25.2
N$26
  Top 0.254: 64.73,24.73 64.73,16.23 63.23,14.73 K6.9 | 64.73,24.73 64.23,25.23 D6.A 64.73,24.73 | 64.73,24.73 65.48,25.48 69.23,25.48 T6.3
N$27
  Top 0.254: T7.2 75.98,26.73 74.48,28.23 74.48,29.98 75.48,30.98 75.48,41.73 R26.2
  Bottom 0.254: R27.2 77.98,41.98 75.73,41.98 R26.2
N$28
  Top 0.254: 73.73,21.23 73.73,24.73 73.23,25.23 D7.A | 73.73,21.23 73.73,16.48 71.98,14.73 K7.9 | 73.73,21.23 77.98,25.48 T7.3
N$29
  Top 0.254: T8.2 84.98,26.73 80.73,30.98 80.73,38.23 84.23,41.73 R28.2
  Bottom 0.254: R29.2 86.98,41.98 84.48,41.98 R28.2
N$30
  Top 0.254: 82.48,24.73 82.48,16.23 80.98,14.73 K8.9 | 82.48,24.73 81.98,25.23 D8.A 82.48,24.73 | 82.48,24.73 83.23,25.48 86.98,25.48 T8.3
NOTAUS  (via drill 0.61)
  Top 0.254: v41.48,43.98 36.73,48.73 34.73,48.73 30.73,52.73 27.98,52.73 NOR#1.4 | v57.98,46.48 v55.48,43.98 | v87.98,62.48 88.48,62.98 88.48,67.23 v88.73,67.48
  Bottom 0.254: v55.48,43.98 v41.48,43.98 | v57.98,46.48 64.73,46.48 67.23,48.98 70.23,48.98 72.73,51.48 75.23,51.48 80.23,56.48 81.98,56.48 v87.98,62.48 | v88.73,67.48 85.98,70.23 85.48,70.23 84.48,71.23 83.73,71.23 RASPBERRY_PI.6
NOTAUS_RAW  (via drill 0.61)
  Top 0.254: NOR#1.6 27.98,47.73 27.98,49.98 NOR#1.5 | v13.98,30.48 14.48,29.98 14.48,23.48 13.98,22.98 TASTER.9 | v15.98,32.48 15.98,36.48 18.23,38.73 v18.23,39.48
  Bottom 0.254: R5.2 39.23,49.73 38.48,48.98 28.98,48.98 27.98,49.98 NOR#1.5 | v15.98,32.48 v13.98,30.48 | v18.23,39.48 26.23,47.48 27.73,47.48 NOR#1.6
RELAIS#1_ENABLE  (via drill 0.61)
  Top 0.254: R14.1 22.23,29.23 20.23,27.23 19.23,27.23 18.23,26.23 18.23,24.23 15.73,21.73 15.73,20.48 15.23,19.98 15.23,15.73 16.73,14.23 16.73,13.73 13.73,10.73 8.23,10.73 6.48,12.48 STATUS_LEDS.1 | v58.48,53.48 58.73,53.48 60.48,55.23 74LS08#1.3 | v57.23,49.73 52.48,44.98 52.48,44.48 50.98,42.98 48.48,42.98 v39.98,34.48
  Bottom 0.254: v58.48,53.48 56.48,51.48 56.48,50.48 v57.23,49.73 | v39.98,34.48 37.73,32.23 25.23,32.23 22.48,29.48 R14.1
RELAIS#1_OUT
  Top 0.254: K1.10 18.48,11.98 12.98,6.48 12.98,5.23 VENTIL#1.1
RELAIS#2_ENABLE  (via drill 0.61)
  Top 0.254: v21.23,21.23 21.23,22.23 22.48,23.48 24.23,23.48 27.98,27.23 28.98,27.23 30.98,29.23 R16.1 | v39.98,31.48 47.48,38.98 51.73,38.98 60.48,47.73 74LS08#1.6
  Bottom 0.254: v21.23,21.23 19.48,19.48 17.23,19.48 14.23,16.48 9.23,16.48 6.73,13.98 5.23,13.98 3.98,12.73 STATUS_LEDS.2 | v39.98,31.48 38.98,30.48 32.23,30.48 31.23,29.48 R16.1
RELAIS#2_OUT
  Top 0.254: K2.10 27.23,11.98 22.98,7.73 22.98,5.23 VENTIL#2.1
RELAIS#3_ENABLE  (via drill 0.61)  (1 unrouted)
  Top 0.254: v44.48,33.73 40.23,29.48 R18.1 | v48.98,34.73 58.23,43.98 61.73,43.98 66.48,48.73 66.48,50.98 67.98,52.48 | v17.48,18.48 v16.23,19.73 | v31.48,18.98 34.48,21.98 34.48,24.73 35.98,26.23 v35.98,28.98
  Bottom 0.254: v44.48,33.73 47.98,33.73 v48.98,34.73 | v16.23,19.73 15.48,18.98 9.98,18.98 6.48,15.48 STATUS_LEDS.3 | v17.48,18.48 17.98,18.98 v31.48,18.98 | v35.98,28.98 36.23,29.23 39.98,29.23 R18.1
RELAIS#3_OUT
  Top 0.254: K3.10 36.23,11.98 33.23,8.98 33.23,5.23 VENTIL#3.1
RELAIS#4_ENABLE  (via drill 0.61)  (1 unrouted)
  Top 0.254: v59.23,37.48 55.48,33.73 53.48,33.73 48.98,29.23 R20.1 | v21.48,23.73 24.73,26.98 25.23,26.98 v29.48,31.23
  Bottom 0.254: v59.23,37.48 66.73,44.98 67.98,44.98 | v21.48,23.73 17.73,23.73 15.73,21.73 11.23,21.73 10.23,20.73 10.23,19.98 6.73,16.48 5.98,16.48 5.48,15.98 4.48,15.98 3.98,15.48 STATUS_LEDS.4 | v29.48,31.23 29.98,31.73 38.98,31.73 39.73,32.48 45.73,32.48 48.73,29.48 R20.1
RELAIS#4_OUT
  Top 0.254: K4.10 45.23,11.98 43.23,9.98 43.23,5.23 VENTIL#4.1
RELAIS#5_ENABLE  (via drill 0.61)
  Top 0.254: v62.73,36.48 v62.73,34.23 | v68.23,42.98 71.73,46.48 71.73,47.98 72.73,48.98 74.48,48.98 75.23,49.73 75.23,53.23 73.48,54.98 74LS08#2.3 | v18.23,8.98 22.98,13.73 29.48,13.73 32.98,17.23 33.73,17.23 v36.48,19.98 | v48.48,21.23 48.48,22.73 49.98,24.23 51.98,24.23 57.23,29.48 57.73,29.48 R22.1
  Bottom 0.254: v62.73,34.23 57.98,29.48 R22.1 | v62.73,36.48 68.23,41.98 v68.23,42.98 | v18.23,8.98 17.73,9.48 5.48,9.48 2.48,12.48 2.48,15.48 3.48,16.48 4.98,16.48 6.23,17.73 STATUS_LEDS.5 | v36.48,19.98 37.73,21.23 v48.48,21.23
RELAIS#5_OUT
  Top 0.254: K5.10 53.98,11.98 53.48,11.48 53.48,5.23 VENTIL#5.1
RELAIS#6_ENABLE  (via drill 0.61)
  Top 0.254: v71.48,34.23 71.73,34.48 71.73,45.73 73.23,47.23 73.23,47.48 74LS08#2.6 | v12.73,11.73 12.48,11.48 10.98,11.48 10.23,12.23 10.23,12.98 6.73,16.48 5.48,16.48 3.98,17.98 STATUS_LEDS.6 | v54.23,20.73 v47.23,13.73 | v56.98,21.23 57.48,21.73 57.48,22.73 58.98,24.23 60.73,24.23 65.98,29.48 66.48,29.48 R24.1
  Bottom 0.254: v71.48,34.23 66.73,29.48 R24.1 | v12.73,11.73 13.48,10.98 37.98,10.98 40.73,13.73 v47.23,13.73 | v54.23,20.73 54.73,21.23 v56.98,21.23
RELAIS#6_OUT
  Top 0.254: K6.10 63.23,11.98 63.48,11.73 63.48,5.23 VENTIL#6.1
RELAIS#7_ENABLE  (via drill 0.61)
  Top 0.254: R26.1 75.73,29.48 78.73,32.48 78.73,40.98 80.98,43.23 80.98,44.98 74LS08#2.8 | v15.73,13.98 10.98,13.98 10.23,14.73 10.23,16.48 6.48,20.23 STATUS_LEDS.7 | v65.73,21.23 66.23,21.73 66.23,22.73 67.73,24.23 69.48,24.23 73.48,28.23 v73.48,28.98
  Bottom 0.254: v15.73,13.98 17.98,16.23 46.98,16.23 49.98,19.23 63.73,19.23 v65.73,21.23 | v73.48,28.98 73.73,29.23 75.48,29.23 R26.1
RELAIS#7_OUT
  Top 0.254: K7.10 71.98,11.98 73.48,10.48 73.48,5.23 VENTIL#7.1
RELAIS#8_ENABLE  (via drill 0.61)
  Top 0.254: v79.73,33.98 80.23,34.48 80.23,41.73 82.73,44.23 82.73,50.98 81.23,52.48 74LS08#2.11 | v8.98,11.73 6.73,13.98 5.98,13.98 5.23,14.73 5.23,15.48 4.23,16.48 3.48,16.48 2.48,17.48 2.48,18.98 3.73,20.23 STATUS_LEDS.8 | v28.23,9.98 31.98,13.73 37.48,13.73 v43.48,19.73 | v74.48,31.23 v70.23,26.98
  Bottom 0.254: R28.1 84.23,29.48 v79.73,33.98 77.23,33.98 v74.48,31.23 | v8.98,11.73 10.73,9.98 v28.23,9.98 | v43.48,19.73 58.73,19.73 61.23,22.23 61.23,22.73 62.23,23.73 65.98,23.73 69.23,26.98 v70.23,26.98
RELAIS#8_OUT
  Top 0.254: K8.10 80.98,11.98 83.73,9.23 83.73,5.23 VENTIL#8.1
RPI_STILL_ALIVE  (via drill 0.61)
  Top 0.254: 79.23,51.73 79.23,53.23 80.98,54.98 74LS08#2.12 | 79.23,51.73 79.23,49.48 80.98,47.73 74LS08#2.9 | 79.23,51.73 73.48,57.48 74LS08#2.2 | 74LS08#2.5 73.23,50.23 68.23,55.23 74LS08#1.12 | v19.73,47.23 15.48,51.48 IC1.3 | 74LS08#1.5 60.48,50.23 v56.98,53.73 56.98,54.23 60.48,57.73 74LS08#1.2
  Bottom 0.254: 74LS08#1.9 68.23,47.73 68.98,48.48 71.73,48.48 73.23,49.98 74LS08#2.5 | 74LS08#2.2 73.23,57.48 71.73,55.98 68.73,55.98 68.23,55.48 74LS08#1.12 67.98,55.48 63.23,55.48 60.98,57.73 60.73,57.73 74LS08#1.2 | v19.73,47.23 26.23,53.73 v56.98,53.73
TASTE#1  (via drill 0.61)
  Top 0.254: v6.98,58.98 2.73,54.73 MCP23008#2.10 | v22.98,57.98 21.73,56.73 21.73,51.23 v26.48,46.48 | v25.23,45.23 30.48,39.98 30.48,30.98 v25.98,26.48 | v25.48,21.23 20.73,16.48 v20.73,14.73
  Bottom 0.254: v6.98,58.98 7.23,58.73 22.23,58.73 v22.98,57.98 | v25.23,45.23 v26.48,46.48 | v25.98,26.48 25.98,22.98 25.48,22.48 v25.48,21.23 | v20.73,14.73 19.23,13.23 16.23,13.23 15.73,12.73 13.98,12.73 TASTER.1
TASTE#2  (via drill 0.61)
  Top 0.254: v8.23,57.73 5.23,54.73 MCP23008#2.11 | v22.98,56.73 26.23,53.48 26.23,52.23 27.23,51.23 28.98,51.23 32.48,47.73 32.48,33.73 38.48,27.73 38.48,22.23 37.23,20.98 36.23,20.98 v33.48,18.23
  Bottom 0.254: v8.23,57.73 9.23,56.73 v22.98,56.73 | v33.48,18.23 31.98,16.73 17.23,16.73 14.48,13.98 13.23,13.98 11.98,12.73 11.48,12.73 TASTER.2
TASTE#3  (via drill 0.61)
  Top 0.254: v2.23,25.48 1.98,25.23 1.98,15.48 3.48,13.98 4.23,13.98 5.23,12.98 5.23,11.73 v6.48,10.48
  Bottom 0.254: v2.23,25.48 1.48,26.23 1.48,38.73 4.98,42.23 5.23,42.23 8.98,45.98 8.98,49.73 7.73,50.98 7.73,54.48 MCP23008#2.12 | v6.48,10.48 9.98,13.98 12.48,13.98 13.73,15.23 TASTER.3
TASTE#4  (via drill 0.61)
  Top 0.254: v9.23,15.23 9.23,16.48 6.73,18.98 5.98,18.98 5.23,19.73 5.23,25.98 1.48,29.73 1.48,38.73 4.98,42.23 5.23,42.23 8.98,45.98 8.98,53.23 10.23,54.48 MCP23008#2.13
  Bottom 0.254: v9.23,15.23 11.23,15.23 TASTER.4
TASTE#5
  Top 0.254: MCP23008#2.14 12.73,54.48 10.48,52.23 10.48,26.23 9.23,24.98 9.23,18.23 10.98,16.48 12.48,16.48 13.73,17.73 TASTER.5
TASTE#6  (via drill 0.61)
  Top 0.254: v13.73,48.48 13.73,52.98 15.23,54.48 MCP23008#2.15 | v9.48,44.23 9.98,43.73 9.98,26.98 v8.98,25.98 | v10.23,24.73 9.73,24.23 9.73,19.48 TASTER.6
  Bottom 0.254: v9.48,44.23 v13.73,48.48 | v10.23,24.73 v8.98,25.98
TASTE#7  (via drill 0.61)
  Top 0.254: v15.98,49.48 11.48,44.98 v11.48,28.73 | v15.48,22.98 15.23,22.73 15.23,21.73 13.98,20.48 TASTER.7
  Bottom 0.254: v15.98,49.48 16.48,49.98 16.48,52.98 17.98,54.48 MCP23008#2.16 | v11.48,28.73 10.73,27.98 10.73,27.23 13.98,23.98 14.48,23.98 v15.48,22.98
TASTE#8  (via drill 0.61)
  Top 0.254: v18.23,32.23 18.23,36.23 19.73,37.73 19.73,40.98 21.48,42.73 21.48,47.48 19.23,49.73 19.23,52.48 19.48,52.73 19.48,53.73 20.23,54.48 MCP23008#2.17 | v12.23,27.73 11.23,26.73 11.23,24.23 10.23,23.23 10.23,21.48 11.23,20.48 TASTER.8
  Bottom 0.254: v18.23,32.23 13.73,27.73 v12.23,27.73
(copper drawn outside any net)
  shapes: Bottom area x2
